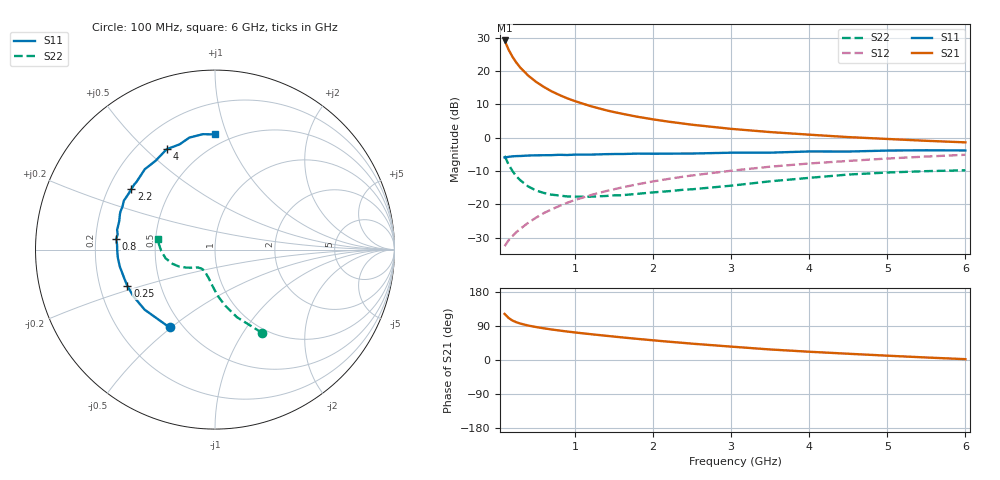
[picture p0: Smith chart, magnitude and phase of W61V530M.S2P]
! SIEMENS Small Signal Semiconductors
! BFR193W
! Si NPN RF Bipolar Junction Transistor in SOT323
! VCE = 1.5 V  IC = 30 mA
! Common Emitter S-Parameters:  September  1992
# GHz  S  MA  R  50
!  f  S11  S21  S12  S22
! GHz  MAG  ANG  MAG  ANG  MAG  ANG  MAG  ANG
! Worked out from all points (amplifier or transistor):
!   28 points, 100 MHz to 6 GHz, reference 50 ohm
!   highest |S21| = 29.2 dB at 100 MHz (marker M1)
!   |S21| within 3 dB of that: start of sweep to 156.6 MHz
!   unconditionally stable (mu >= 1): 577.3 MHz to 2.578 GHz
!   at 300 MHz: K = 0.87, MSG = 24.2 dB, |S12| = -27.4 dB
!   at 1.5 GHz: K = 1.04, MAG = 10.4 dB, |S12| = -15.5 dB
!   at 6 GHz: K = 0.93, MSG = 1.9 dB, |S12| = -5.1 dB
!   S11 on the Smith chart (normalised r, x): 100 MHz: 0.42, -0.49; 250 MHz: 0.32, -0.18; 800 MHz: 0.29, +0.05; 2.2 GHz: 0.30, +0.30; 4 GHz: 0.32, +0.58; 6 GHz: 0.42, +0.91
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0.1  0.5024 -120.3  28.79 121.7  0.0235 56.8  0.5333 -60.5
0.15  0.5155 -139.5  21.05 111.0  0.0287 56.4  0.3961 -72.0
0.2  0.5241 -150.3  16.43 104.2  0.0332 58.1  0.3169 -79.7
0.25  0.5286 -157.5  13.41 99.7  0.0381 60.0  0.2636 -85.9
0.3  0.5303 -162.6  11.31 96.2  0.0427 62.1  0.2301 -89.9
0.4  0.5389 -170.0  8.583 91.0  0.0525 65.2  0.1859 -97.2
0.5  0.5433 -175.3  6.921 87.1  0.0627 67.0  0.1614 -102.8
0.6  0.5448 -179.5  5.798 83.7  0.0735 68.2  0.1482 -108.1
0.7  0.5463 177.1  4.97 80.6  0.0837 69.1  0.1395 -111.8
0.8  0.5534 174.0  4.378 77.8  0.0942 69.5  0.1354 -115.3
0.9  0.5491 171.1  3.899 75.2  0.1052 69.5  0.1311 -118.2
1  0.5563 168.6  3.539 72.7  0.1158 69.4  0.1303 -120.5
1.2  0.5566 163.5  2.976 68.2  0.137 68.8  0.1301 -126.2
1.4  0.5654 159.5  2.577 63.9  0.1578 67.9  0.1332 -129.7
1.6  0.568 155.3  2.291 59.7  0.1788 66.9  0.1368 -133.3
2.2  0.5749 144.1  1.738 48.3  0.2405 62.6  0.1571 -140.1
3  0.5946 131.1  1.356 35.3  0.319 55.9  0.1902 -148.2
3.5  0.5954 123.8  1.213 27.8  0.3665 51.4  0.2211 -154.7
4  0.6207 115.7  1.109 21.8  0.4095 46.8  0.2492 -161.4
4.5  0.6186 108.6  1.02 16.5  0.4475 42.4  0.2794 -170.0
5.5  0.6466 96.1  0.897 6.6  0.5206 33.6  0.3143 174.3
6  0.642 89.8  0.85 2.2  0.5537 29.0  0.3236 169.6
